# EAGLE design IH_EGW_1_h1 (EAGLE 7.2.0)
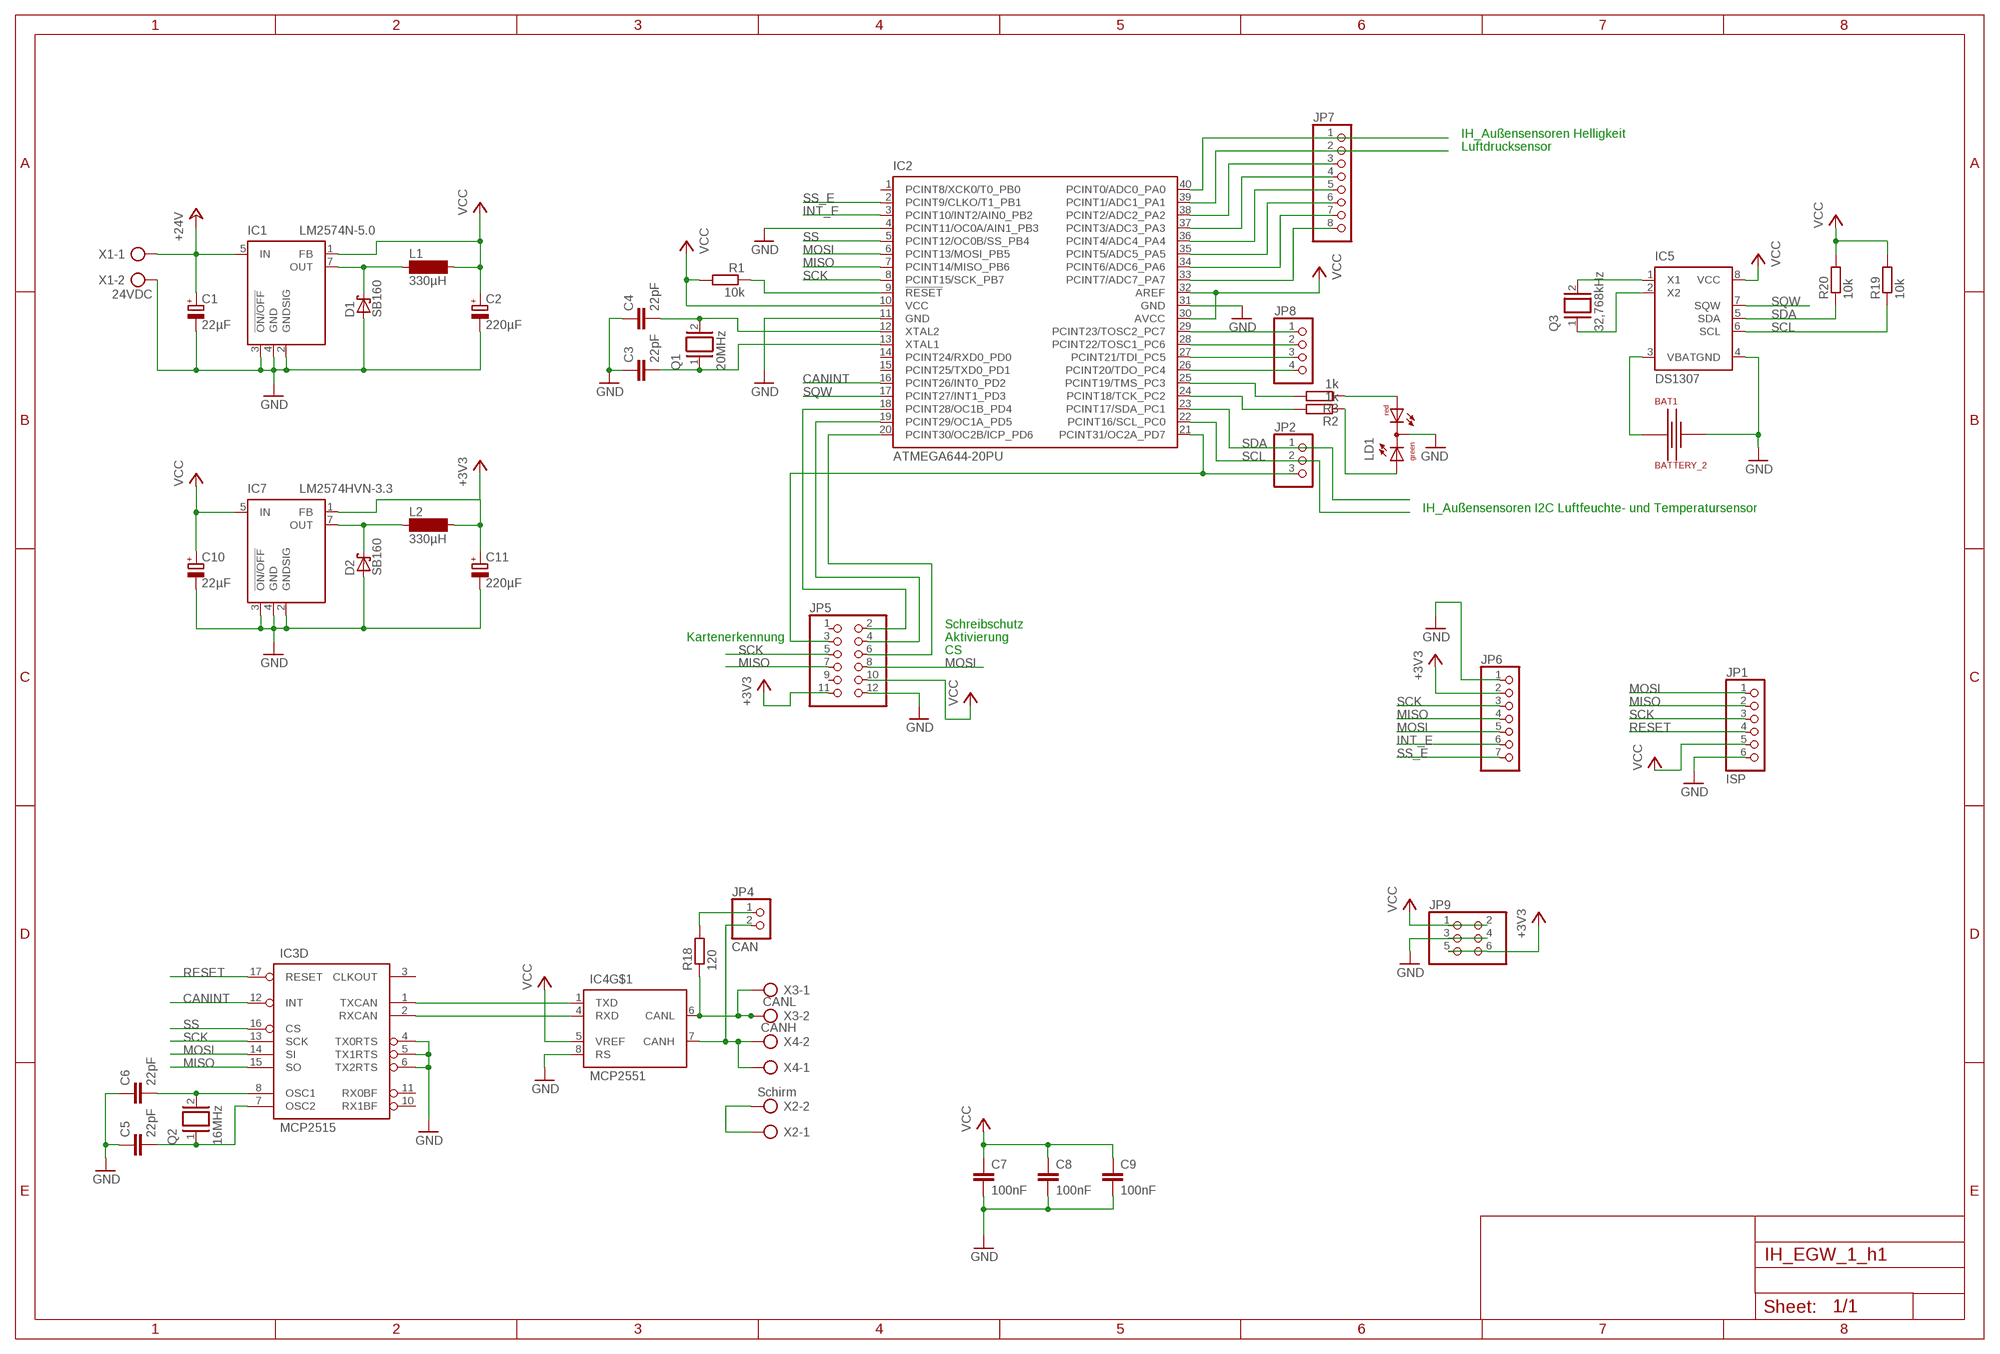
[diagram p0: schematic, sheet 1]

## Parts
BAT1  BATTERY_2  [BATTERY_2]
C1  22µF  CPOL-EUE2-5  [E2-5]
C2  220µF  CPOL-EUE3.5-8  [E3,5-8]
C3  22pF  C-EUC0805  [C0805]
C4  22pF  C-EUC0805  [C0805]
C5  22pF  C-EUC0805  [C0805]
C6  22pF  C-EUC0805  [C0805]
C7  100nF  C-EUC0805  [C0805]
C8  100nF  C-EUC0805  [C0805]
C9  100nF  C-EUC0805  [C0805]
C10  22µF  CPOL-EUE2-5  [E2-5]
C11  220µF  CPOL-EUE3.5-8  [E3,5-8]
D1  SB160  SCHOTTKY-DIODEDO35-7  [DO35-7]
D2  SB160  SCHOTTKY-DIODEDO35-7  [DO35-7]
IC1  LM2574N-5.0  [DIL08]
IC2  ATMEGA644-20PU  [DIL40]
IC3  MCP2515  MCP2515P  [DIL18]
IC4  MCP2551  MCP2551DIL8  [DIL08]
IC5  DS1307  [DIP-8]
IC7  LM2574HVN-3.3  [DIL08]
JP1  ISP  PINHD-1X6  [1X06]
JP2  PINHD-1X3  [1X03]
JP4  CAN  PINHD-1X2  [1X02]
JP5  PINHD-2X6  [2X06]
JP6  PINHD-1X7  [1X07]
JP7  PINHD-1X8  [1X08]
JP8  PINHD-1X4  [1X04]
JP9  PINHD-2X3  [2X03]
L1  330µH  SD12-1000  [SD12_1000]
L2  330µH  SD12-1000  [SD12_1000]
LD1  DUOLED-RG-C  [DUOLED-C-5MM]
Q1  20MHz  XTAL/S  [QS]
Q2  16MHz  XTAL/S  [QS]
Q3  32,768kHz  XTAL/S  [QS]
R1  10k  R-EU_R0805  [R0805]
R2  1k  R-EU_M0805  [M0805]
R3  1k  R-EU_M0805  [M0805]
R18  120  R-EU_M0805  [M0805]
R19  10k  R-EU_M0805  [M0805]
R20  10k  R-EU_M0805  [M0805]
X1  24VDC  AK300/2  [AK300/2]
X2  Schirm  AK300/2  [AK300/2]
X3  CANL  AK300/2  [AK300/2]
X4  CANH  AK300/2  [AK300/2]

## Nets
+3V3: C11.+ IC7.1(FB) JP5.11 JP6.2 JP9.5 JP9.6 L2.2
+24V: C1.+ IC1.5(IN) X1.1
CANINT: IC2.16(PCINT26/INT0_PD2) IC3.12(D:INT)
GND: BAT1.P$2(-) C1.- C2.- C3.1 C4.1 C5.1 C6.1 C7.2 C8.2 C9.2 C10.- C11.- D1.A D2.A IC1.2(GNDSIG) IC1.3(!ON/OFF) IC1.4(GND) IC2.4(PCINT11/OC0A/AIN1_PB3) IC2.11(GND) IC2.31(GND) IC3.4(D:TX0RTS) IC3.5(D:TX1RTS) IC3.6(D:TX2RTS) IC4.8(RS) IC5.4(GND) IC7.2(GNDSIG) IC7.3(!ON/OFF) IC7.4(GND) JP1.6 JP5.12 JP6.1 JP9.3 JP9.4 LD1.C X1.2
INT_E: IC2.3(PCINT10/INT2/AIN0_PB2) JP6.6
MISO: IC2.7(PCINT14/MISO_PB6) IC3.15(D:SO) JP1.2 JP5.7 JP6.4
MOSI: IC2.6(PCINT13/MOSI_PB5) IC3.14(D:SI) JP1.1 JP5.8 JP6.5
N$1: IC3.1(D:TXCAN) IC4.1(TXD)
N$2: IC3.2(D:RXCAN) IC4.4(RXD)
N$3: C6.2 IC3.8(D:OSC1) Q2.2
N$4: C5.2 IC3.7(D:OSC2) Q2.1
N$7: C4.2 IC2.12(XTAL2) Q1.2
N$8: C3.2 IC2.13(XTAL1) Q1.1
N$9: IC2.33(PCINT7/ADC7_PA7) JP7.8
N$10: IC2.34(PCINT6/ADC6_PA6) JP7.7
N$11: IC2.35(PCINT5/ADC5_PA5) JP7.6
N$12: IC2.36(PCINT4/ADC4_PA4) JP7.5
N$13: IC2.37(PCINT3/ADC3_PA3) JP7.4
N$14: IC2.38(PCINT2/ADC2_PA2) JP7.3
N$15: IC2.39(PCINT1/ADC1_PA1) JP7.2
N$16: IC4.6(CANL) R18.1 X3.1 X3.2
N$17: IC4.7(CANH) JP4.2 X4.1 X4.2
N$18: IC2.40(PCINT0/ADC0_PA0) JP7.1
N$19: IC2.29(PCINT23/TOSC2_PC7) JP8.1
N$20: IC2.20(PCINT30/OC2B/ICP_PD6) JP5.6
N$22: IC2.19(PCINT29/OC1A_PD5) JP5.4
N$23: IC2.18(PCINT28/OC1B_PD4) JP5.2
N$24: IC2.28(PCINT22/TOSC1_PC6) JP8.2
N$25: IC2.27(PCINT21/TDI_PC5) JP8.3
N$26: IC2.25(PCINT19/TMS_PC3) R3.2
N$27: D2.C IC7.7(OUT) L2.1
N$28: IC2.26(PCINT20/TDO_PC4) JP8.4
N$29: BAT1.P$1(+) IC5.3(VBAT)
N$30: IC2.21(PCINT31/OC2A_PD7) JP2.3 JP5.3
N$31: IC5.1(X1) Q3.2
N$32: IC5.2(X2) Q3.1
N$33: IC2.24(PCINT18/TCK_PC2) R2.2
N$42: LD1.AX(AG) R2.1
N$43: LD1.AR R3.1
N$44: JP4.1 R18.2
N$54: X2.1 X2.2
N$76: D1.C IC1.7(OUT) L1.1
RESET: IC2.9(!RESET) IC3.17(D:RESET) JP1.4 R1.1
SCK: IC2.8(PCINT15/SCK_PB7) IC3.13(D:SCK) JP1.3 JP5.5 JP6.3
SCL: IC2.22(PCINT16/SCL_PC0) IC5.6(SCL) JP2.2 R19.1
SDA: IC2.23(PCINT17/SDA_PC1) IC5.5(SDA) JP2.1 R20.1
SQW: IC2.17(PCINT27/INT1_PD3) IC5.7(SQW)
SS: IC2.5(PCINT12/OC0B/SS_PB4) IC3.16(D:CS)
SS_E: IC2.2(PCINT9/CLKO/T1_PB1) JP6.7
VCC: C2.+ C7.1 C8.1 C9.1 C10.+ IC1.1(FB) IC2.10(VCC) IC2.30(AVCC) IC2.32(AREF) IC4.5(VREF) IC5.8(VCC) IC7.5(IN) JP1.5 JP5.10 JP9.1 JP9.2 L1.2 R1.2 R19.2 R20.2
Unconnected: IC2.1(PCINT8/XCK0/T0_PB0) IC2.14(PCINT24/RXD0_PD0) IC2.15(PCINT25/TXD0_PD1) IC3.3(D:CLKOUT) IC3.10(D:RX1BF) IC3.11(D:RX0BF) JP5.1 JP5.9

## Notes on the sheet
- IH_Außensensoren Helligkeit
- Luftdrucksensor
- IH_Außensensoren I2C Luftfeuchte- und Temperatursensor
- Schreibschutz
- Kartenerkennung | Aktivierung
- CS

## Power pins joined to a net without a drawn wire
GND: IC3.9(P:GND) IC4.2(GND)
VCC: IC3.18(P:VCC) IC4.3(VCC)

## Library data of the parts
BAT1 = special:BATTERY_2
C1 C2 C10 C11 = rcl:CPOL-EU: POLARIZED CAPACITOR, European symbol
C3-C9 = rcl:C-EU: CAPACITOR, European symbol
D1 D2 = diode:SCHOTTKY-DIODE: Schottky Diode
IC1 IC7 = linear:LM2574?-*: SIMPLE SWITCHER 0.5A Step-Down Voltage Regulator Source: http://cache.national.com/ds/LM/LM2574.pdf
IC2 = atmel:ATMEGA644-*PU: 8-bit Microcontroller with 64K Bytes In-System Programmable Flash Auto generated by make-symbol-device-package-bsdl.ulp Rev. 34 Source: http://www.atmel.com/dyn/resources/prod_documents/doc2593.pdf; MPN: ATMEGA644-20PU; OC_FARNELL: 1288340; OC_NEWARK: 23M5060
IC3 = can:MCP2515: MC2515 Stand-Alone CAN Controller With SPI Interface, Microchip
IC4 = can:MCP2551: CAN Tranceiver Microchip
IC5 = DS1307:DS1307: DS1307 - 64×8, Serial, I2C Real Time Clock
JP1 = pinhead:PINHD-1X6: PIN HEADER
JP2 = pinhead:PINHD-1X3: PIN HEADER
JP4 = pinhead:PINHD-1X2: PIN HEADER
JP5 = pinhead:PINHD-2X6: PIN HEADER
JP6 = pinhead:PINHD-1X7: PIN HEADER
JP7 = pinhead:PINHD-1X8: PIN HEADER
JP8 = pinhead:PINHD-1X4: PIN HEADER
JP9 = pinhead:PINHD-2X3: PIN HEADER
L1 L2 = inductor-neosid:SD12: INDUCTOR; OC_FARNELL: unknown; OC_NEWARK: unknown
LD1 = led:DUOLED-RG-C: DUO LED 2 colors (red/green), 5 mm, round, common Cathode www.ligitek.com or other producers.
Q1-Q3 = special:XTAL/S: CRYSTAL
R1 R18 = rcl:R-EU_: RESISTOR, European symbol
R2 R3 R19 R20 = resistor:R-EU_: RESISTOR, European symbol
X1-X4 = con-ptr500:AK300/2: CONNECTOR; OC_FARNELL: unknown; OC_NEWARK: unknown

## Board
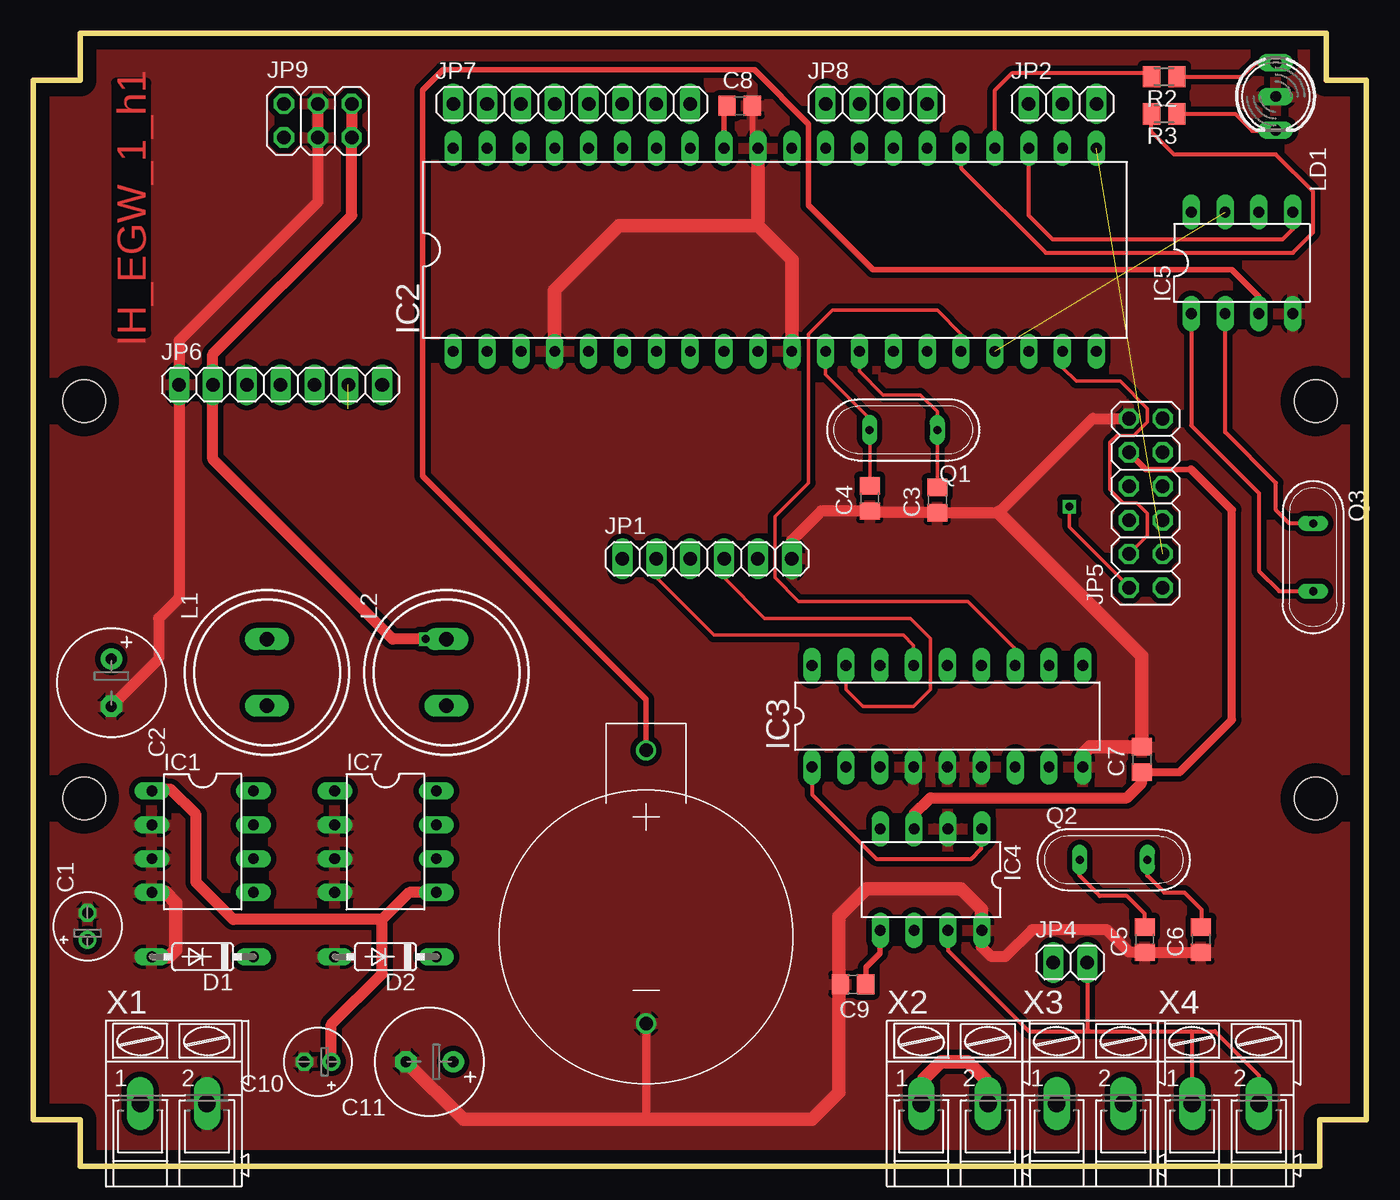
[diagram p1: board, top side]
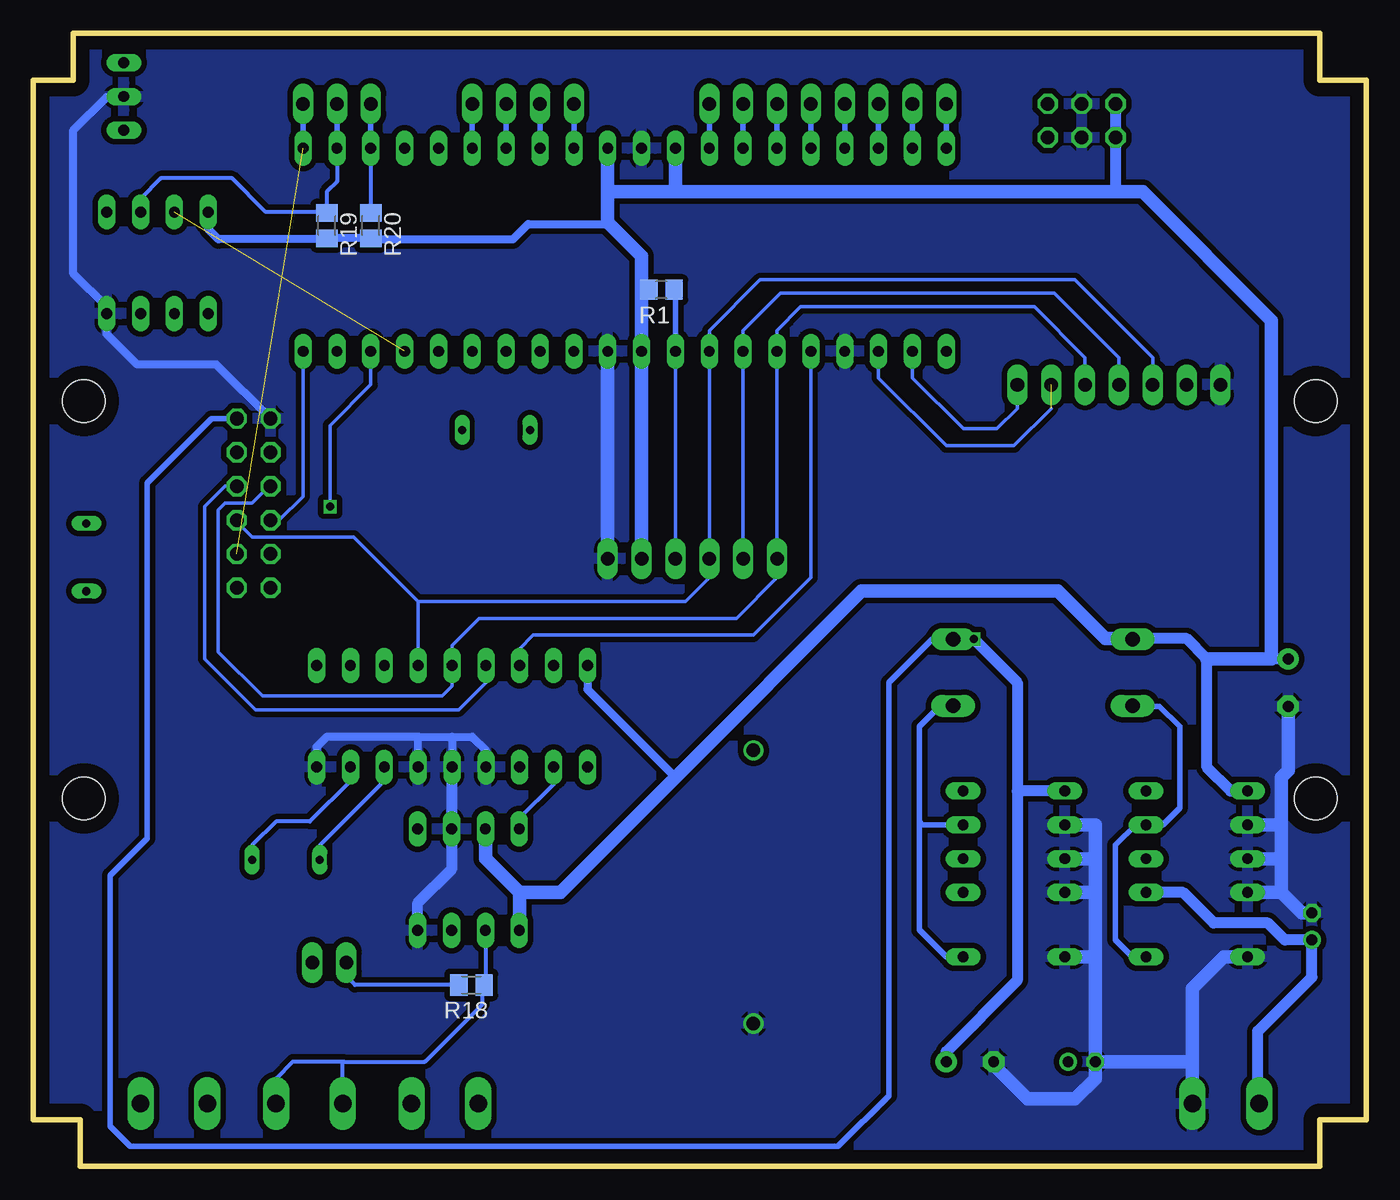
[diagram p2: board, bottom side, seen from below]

Size 100 x 85 mm. Coordinates in mm from the lower left corner, seen from the top.
Outline: 100,3.5 100,80
Outline: 0,80 0,3.5
Outline: 0,3.5 3.5,3.5 3.5,0 96.5,0 96.5,3.5 100,3.5
Outline: 0,3.5 0,81.5 3.5,81.5 3.5,85 97,85 97,81.5 100,81.5 100,3.5
Copper layers (1*16): Top 0.035mm / dielectric 1.5mm / Bottom 0.035mm
Design rules "default *": minimum track width 10mil, minimum drill 36mil, track to track 15mil, track to pad 15mil, pad to pad 10mil, via to via 10mil, smd to smd 10mil, copper to edge 40mil, drill to drill 8mil, minimum pad ring 10mil, minimum via ring 8mil, stop-mask expansion 4mil, vias tented up to drill 0mil, thermal gap 10mil
Holes 3.2 mm at 3.8,27.6 3.8,57.4 96.2,27.6 96.2,57.4

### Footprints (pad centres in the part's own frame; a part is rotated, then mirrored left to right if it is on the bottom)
BATTERY_2 = drill 1: P$1 0,0; P$2 0,20.5
E2-5 = drill 0.813 pad 1.27: + -1.016,0 | drill 0.813 pad 1.27 octagon: - 1.016,0
E3,5-8 = drill 0.813 pad 1.6: + -1.778,0 | drill 0.813 pad 1.6 octagon: - 1.778,0
C0805 = smd 1.3 x 1.5: 1 -0.95,0; 2 0.95,0
DO35-7 = drill 0.813 long: A 3.81,0; C -3.81,0
DIL08 = drill 0.813 pad 1.27 long: 1 -3.81,-3.81; 2 -1.27,-3.81; 3 1.27,-3.81; 4 3.81,-3.81; 5 3.81,3.81; 6 1.27,3.81; 7 -1.27,3.81; 8 -3.81,3.81
DIL40 = drill 0.813 long: 1 -24.13,-7.62; 2 -21.59,-7.62; 3 -19.05,-7.62; 4 -16.51,-7.62; 5 -13.97,-7.62; 6 -11.43,-7.62; 7 -8.89,-7.62; 8 -6.35,-7.62; 9 -3.81,-7.62; 10 -1.27,-7.62; 11 1.27,-7.62; 12 3.81,-7.62; 13 6.35,-7.62; 14 8.89,-7.62; 15 11.43,-7.62; 16 13.97,-7.62; 17 16.51,-7.62; 18 19.05,-7.62; 19 21.59,-7.62; 20 24.13,-7.62; 21 24.13,7.62; 22 21.59,7.62; 23 19.05,7.62; 24 16.51,7.62; 25 13.97,7.62; 26 11.43,7.62; 27 8.89,7.62; 28 6.35,7.62; 29 3.81,7.62; 30 1.27,7.62; 31 -1.27,7.62; 32 -3.81,7.62; 33 -6.35,7.62; 34 -8.89,7.62; 35 -11.43,7.62; 36 -13.97,7.62; 37 -16.51,7.62; 38 -19.05,7.62; 39 -21.59,7.62; 40 -24.13,7.62
DIL18 = drill 0.813 long: 1 -10.16,-3.81; 2 -7.62,-3.81; 3 -5.08,-3.81; 4 -2.54,-3.81; 5 0,-3.81; 6 2.54,-3.81; 7 5.08,-3.81; 8 7.62,-3.81; 9 10.16,-3.81; 10 10.16,3.81; 11 7.62,3.81; 12 5.08,3.81; 13 2.54,3.81; 14 0,3.81; 15 -2.54,3.81; 16 -5.08,3.81; 17 -7.62,3.81; 18 -10.16,3.81
DIL08' = drill 0.813 long: 1 -3.81,-3.81; 2 -1.27,-3.81; 3 1.27,-3.81; 4 3.81,-3.81; 5 3.81,3.81; 6 1.27,3.81; 7 -1.27,3.81; 8 -3.81,3.81
DIP-8 = drill 0.813 long: 1 -3.81,-3.81; 2 -1.27,-3.81; 3 1.27,-3.81; 4 3.81,-3.81; 5 3.81,3.81; 6 1.27,3.81; 7 -1.27,3.81; 8 -3.81,3.81
1X06 = drill 1.016 long: 1 -6.35,0; 2 -3.81,0; 3 -1.27,0; 4 1.27,0; 5 3.81,0; 6 6.35,0
1X03 = drill 1.016 long: 1 -2.54,0; 2 0,0; 3 2.54,0
1X02 = drill 1.016 long: 1 -1.27,0; 2 1.27,0
2X06 = drill 1.016 octagon: 1 -6.35,-1.27; 2 -6.35,1.27; 3 -3.81,-1.27; 4 -3.81,1.27; 5 -1.27,-1.27; 6 -1.27,1.27; 7 1.27,-1.27; 8 1.27,1.27; 9 3.81,-1.27; 10 3.81,1.27; 11 6.35,-1.27; 12 6.35,1.27
1X07 = drill 1.016 long: 1 -7.62,0; 2 -5.08,0; 3 -2.54,0; 4 0,0; 5 2.54,0; 6 5.08,0; 7 7.62,0
1X08 = drill 1.016 long: 1 -8.89,0; 2 -6.35,0; 3 -3.81,0; 4 -1.27,0; 5 1.27,0; 6 3.81,0; 7 6.35,0; 8 8.89,0
1X04 = drill 1.016 long: 1 -3.81,0; 2 -1.27,0; 3 1.27,0; 4 3.81,0
2X03 = drill 1.016 octagon: 1 -2.54,-1.27; 2 -2.54,1.27; 3 0,-1.27; 4 0,1.27; 5 2.54,-1.27; 6 2.54,1.27
SD12_1000 = drill 1.1 long: 1 -2.5,0; 2 2.5,0
DUOLED-C-5MM = drill 0.813 long: AR 2.54,0; AX -2.54,0; C 0,0
QS = drill 0.61 long: 1 -2.54,0; 2 2.54,0
R0805 = smd 1.3 x 1.5: 1 -0.95,0; 2 0.95,0
M0805 = smd 1.3 x 1.6: 1 -0.95,0; 2 0.95,0
AK300/2 = drill 1.321 long: 1 -2.515,0; 2 2.489,0

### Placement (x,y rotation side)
BAT1  45.98,31.2 180 top
C1  4.07,17.99 90 top
C2  5.85,36.28 270 top
C3  67.83,49.99 90 top
C4  62.75,50.11 90 top
C5  83.38,17 90 top
C6  87.61,17 90 top
C7  83.17,30.51 90 top
C8  53,79.56 0 top
C9  61.5,13.65 180 top
C10  21.34,7.83 180 top
C11  29.73,7.83 180 top
D1  12.71,15.71 180 top
D2  26.42,15.71 180 top
IC1  12.71,24.34 270 top
IC2  55.63,68.76 0 top
IC3  68.59,33.76 0 top
IC4  MCP2551  [DIL08']  67.35,21.5 180 top
IC5  90.69,67.78 0 top
IC7  26.42,24.34 270 top
JP1  50.55,45.58 0 top
JP2  77.22,79.72 0 top
JP4  77.79,15.28 0 top
JP5  83.47,49.74 90 top
JP6  18.55,58.63 0 top
JP7  40.39,79.72 0 top
JP8  63.25,79.72 0 top
JP9  21.34,78.45 0 top
L1  17.53,37.04 90 top
L2  31,37.04 90 top
LD1  93.21,80.26 270 top
Q1  65.28,55.24 180 top
Q2  81.05,22.99 0 top
Q3  96.02,45.68 270 top
R1  52.88,65.76 180 bottom
R2  84.84,81.75 180 top
R3  84.84,78.95 180 top
R18  67.13,13.59 180 bottom
R19  77.99,70.57 270 bottom
R20  74.68,70.57 270 bottom
X1  10.54,4.7 0 top
X2  69.14,4.7 0 top
X3  79.3,4.7 0 top
X4  89.46,4.7 0 top

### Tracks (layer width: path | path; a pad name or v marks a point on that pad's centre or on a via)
+3V3  (via drill 0.6)
  Top 0.813: v29.43,39.54 26.97,39.54 13.47,53.05 JP6.2 13.47,60.92 23.88,71.33 JP9.5 JP9.6
  Bottom 0.406: L2.2 32.56,39.54 35.82,36.28 35.82,5.29 39.63,1.48 92.72,1.48 94.24,3.01 94.24,21.8 91.45,24.6 91.45,51.27 86.62,56.09 JP5.11
  Bottom 0.813: C11.+ 31.5,8.6 26.17,13.93 26.17,28.15 | IC7.1 26.17,28.15 | L2.2 v29.43,39.54 26.17,36.28 26.17,28.15
+24V
  Bottom 0.813: X1.1 8.14,4.7 8.14,10.12 4.07,14.18 C1.+ 6.1,16.98 7.37,18.25 11.44,18.25 13.72,20.53 IC1.5
CANINT
  Top 0.254: IC3.12 73.67,38.82 70.11,42.38 57.41,42.38 55.63,44.16 55.63,48.73 58.17,51.27 58.17,62.44 59.95,64.22 67.83,64.22 69.6,62.44 IC2.16
GND
  Top 0.406: C9.2 60.55,15.36 60.46,15.45 | IC2.31 53.95,76.8 C8.2
  Top 0.61: BAT1.P$2 45.98,3.52
  Top 0.813: JP5.12 79.51,56.09 72.45,49.04 72.4,49.04 C3.1 62.87,49.04 C4.1 59.11,49.16 56.9,46.95 JP1.6 | C6.1 C5.1 82.22,16.05 80.53,17.74 74.94,17.74 72.91,15.71 71.89,15.71 71.13,16.47 71.13,17.66 IC4.8 | C2.- 9.41,38.06 9.41,41.11 10.93,42.63 JP6.1 10.93,61.94 21.34,72.35 JP9.3 JP9.4
  Top 1.016: IC2.31 54.36,70.57 | 54.36,70.57 56.9,68.03 IC2.11 | IC2.4 39.12,65.75 43.95,70.57 54.36,70.57 | 72.4,49.04 83.17,38.27 C7.2 79.26,31.46 78.75,30.95 IC3.9 | C11.- 32.27,3.52 45.98,3.52 58.43,3.52 60.46,5.55 60.46,15.45 60.46,18.76 62.49,20.79 69.6,20.79 71.13,19.26 71.13,17.99 | IC1.4 9.91,20.53 10.68,19.77 10.68,16.22 10.17,15.71 D1.A
  Bottom 0.406: 68.62,29.95 IC3.5
  Bottom 0.61: IC3.6 71.13,32.22 | 71.13,32.22 68.59,32.22 | 71.13,32.22 77.99,32.22 78.75,31.46 IC3.9 | 68.59,32.22 IC3.5 | 68.59,32.22 67.06,32.22 66.05,31.2 IC3.4 | LD1.C 93.25,80.22 94.5,80.22 97.04,77.68 97.04,67.02 94.5,64.48 IC5.4 94.5,62.44 92.21,60.16 86.26,60.16 JP5.12
  Bottom 0.813: 68.62,29.95 IC4.2 68.59,25.28 68.59,22.31 71.16,19.74 IC4.8
  Bottom 1.016: X1.2 13.03,7.83 | 13.03,7.83 13.03,13.36 10.68,15.71 D1.A | C10.- 13.03,7.83 | C10.- 20.33,15.96 | 20.33,15.96 20.33,20.53 | 20.33,20.53 20.33,23.07 | 20.33,23.07 20.33,25.61 IC7.2 | IC7.3 20.33,23.07 | IC7.4 20.33,20.53 | D2.A 20.58,15.71 20.33,15.96 | C2.- 5.85,29.68 6.36,29.17 6.36,25.61 | 6.36,25.61 6.36,23.07 | 6.36,23.07 6.36,20.79 | 6.36,20.79 6.36,20.53 4.83,19.01 C1.- | IC1.4 6.61,20.53 6.36,20.79 | IC1.3 6.36,23.07 | IC1.2 6.36,25.61 | C11.- 27.95,7.58 25.41,5.04 21.85,5.04 20.33,6.56 C10.- | IC2.11 JP1.6
  pour Bottom (isolate 0.406): -2.79,87.59 101.86,87.59 101.86,-2.83 -3.29,-2.83 -3.29,87.59
  pour Top (isolate 0.406): -2.28,86.83 102.37,86.83 102.37,-2.07 -1.77,-2.07 -1.77,86.57
INT_E  (1 unrouted)
  Bottom 0.254: IC2.3 36.58,59.14 31.5,54.06 26.42,54.06 23.63,56.86
MISO
  Top 0.254: JP1.2 46.74,44.16 51.06,39.84 65.29,39.84 66.05,39.08 IC3.15
  Bottom 0.254: JP1.2 IC2.7 46.74,62.7 43.95,65.49 23.38,65.49 18.55,60.67 JP6.4 | JP5.7 85.61,51.01 87.13,49.49 87.13,38.06 83.32,34.25 68.08,34.25 66.05,36.28 IC3.15
MOSI
  Bottom 0.254: JP5.8 82.3,51.01 83.57,49.74 85.61,49.74 86.11,49.24 86.11,38.57 82.81,35.27 69.35,35.27 68.59,36.03 IC3.14 68.59,39.08 66.56,41.11 47.25,41.11 44.2,44.16 JP1.1 IC2.6 44.2,62.7 42.43,64.48 24.9,64.48 21.09,60.67 JP6.5
N$1
  Top 0.305: IC3.1 58.43,27.9 63.25,23.07 70.37,23.07 71.13,23.84 71.13,25.28 IC4.1
N$2
  Bottom 0.305: IC3.2 60.97,28.66 63.51,26.12 63.51,25.34 IC4.4
N$3
  Top 0.305: Q2.2 83.59,21.82 83.57,21.8 84.84,20.53 86.37,20.53 87.64,19.26 87.64,17.98 C6.2
  Bottom 0.305: IC3.8 76.21,28.92 79.26,25.87 81.8,25.87 83.57,24.09 83.57,23 Q2.2
N$4
  Top 0.305: C5.2 83.38,18.95 82.05,20.28 80.02,20.28 78.49,21.8 78.49,22.98 Q2.1
  Bottom 0.305: IC3.7 73.67,28.92 78.49,24.09 78.49,22.98 | 78.49,22.57 78.49,22.98 | 78.49,22.98 Q2.1
N$6  (via drill 0.6)
  other vias: 77.73,49.49
N$7
  Top 0.254: C4.2 Q1.2 62.75,55.25 62.75,56.09 59.44,59.4 IC2.12
N$8
  Top 0.254: IC2.13 61.98,59.65 63.76,57.87 66.56,57.87 67.83,56.6 67.83,55.25 Q1.1 67.82,50.95 C3.2
N$9
  Bottom 0.406: JP7.8 IC2.33
N$10
  Bottom 0.406: JP7.7 IC2.34
N$11
  Bottom 0.406: JP7.6 IC2.35
N$12
  Bottom 0.406: JP7.5 IC2.36
N$13
  Bottom 0.406: JP7.4 IC2.37
N$14
  Bottom 0.406: JP7.3 IC2.38
N$15
  Bottom 0.406: JP7.2 IC2.39
N$16
  Bottom 0.305: IC4.6 66.08,13.7 R18.1 66.3,13.48 66.3,12.15 70.62,7.83 76.72,7.83 | X3.1 76.78,7.76 76.72,7.83 | 76.72,7.83 80.53,7.83 81.8,6.56 X3.2
N$17
  Top 0.305: IC4.7 68.62,16.18 74.68,10.12 79.26,10.12 | 79.26,10.12 86.88,10.12 | 86.88,10.12 88.65,10.12 91.96,6.82 X4.2 | X4.1 86.94,10.05 86.88,10.12 | JP4.2 79.06,10.31 79.26,10.12
N$18
  Bottom 0.406: JP7.1 IC2.40
N$19
  Bottom 0.406: JP8.1 IC2.29
N$20
  Bottom 0.254: JP5.6 81.54,48.47 79.76,50.25 IC2.20
N$22
  Top 0.254: IC2.19 77.22,59.9 78.24,58.89 81.54,58.89 83.57,56.86 83.57,55.84 82.56,54.82 81.29,54.82 80.78,54.32 80.78,50.76 81.8,49.74 82.81,49.74 83.57,48.98 83.57,47.31 JP5.4
N$23  (via drill 0.6)
  Top 0.254: JP5.2 82.2,43.5 77.73,47.97 v77.73,49.49
  Bottom 0.254: v77.73,49.49 77.73,55.59 74.68,58.63 IC2.18
N$24
  Bottom 0.406: JP8.2 IC2.28
N$25
  Bottom 0.406: JP8.3 IC2.27
N$26
  Top 0.305: IC2.25 69.6,74.89 75.95,68.54 94.5,68.54 96.02,70.06 96.02,73.11 93.23,75.91 85.61,75.91 83.89,77.62 R3.2
N$27
  Bottom 0.406: D2.C 31.5,15.71 33.54,17.74 33.54,25.87 | 33.54,25.87 33.54,32.98 32.01,34.5 31.04,34.5 L2.1 | IC7.7 33.28,25.61 33.54,25.87
N$28
  Bottom 0.406: JP8.4 IC2.26
N$29
  Top 0.406: IC5.3 91.96,65.24 89.92,67.27 63,67.27 58.17,72.1 58.17,78.19 54.11,82.26 30.74,82.26 29.22,80.73 29.22,51.78 45.98,35.01 BAT1.P$1
N$30  (1 unrouted)
  Bottom 0.406: IC2.21 JP2.3
N$31
  Top 0.305: IC5.1 86.88,55.59 91.96,50.51 91.96,44.66 93.48,43.14 Q3.2
N$32
  Top 0.305: Q3.1 94.24,48.22 93.23,49.24 93.23,51.27 89.42,55.08 IC5.2
N$33
  Top 0.305: IC2.24 72.14,80.73 73.41,82 83.64,82 R2.2
N$42
  Top 0.305: R2.1 90.69,81.75 91.7,82.76 93.17,82.76 LD1.AX
N$43
  Top 0.305: R3.1 90.18,78.95 91.45,77.68 93.17,77.68 LD1.AR
N$44
  Bottom 0.305: R18.2 75.87,13.59 76.46,14.18 76.46,15.22 JP4.1
N$54
  Top 1.016: X2.1 66.81,4.7 66.81,6.56 68.08,7.83 70.11,7.83 71.38,6.56 71.38,4.95 X2.2
N$76
  Bottom 0.406: L1.1 17.49,34.5 15.5,34.5 13.98,32.98 13.98,26.88 15.25,25.61 IC1.7 17.28,25.61 18.8,24.09 18.8,16.98 17.53,15.71 D1.C
RESET
  Top 0.254: IC3.17 60.97,35.77 62.24,34.5 66.05,34.5 67.32,35.77 67.32,39.58 65.79,41.11 54.87,41.11 51.82,44.16 JP1.4
  Bottom 0.254: IC2.9 JP1.4
  Bottom 0.406: 51.93,61.24 IC2.9 51.82,65.65 R1.1
SCK
  Bottom 0.254: 71.13,42.38 51.06,42.38 49.28,44.16 JP1.3 IC2.8 49.28,62.7 45.47,66.51 21.85,66.51 16.01,60.67 JP6.3 | JP5.5 84.74,48.37 83.57,47.2 75.95,47.2 71.13,42.38 | IC3.13 71.13,42.38
SCL
  Bottom 0.305: IC2.22 77.22,73.87 77.99,73.11 R19.1 78.05,71.59 82.56,71.59 85.1,74.13 90.43,74.13 91.96,72.6 IC5.6
  Bottom 0.406: JP2.2 IC2.22
SDA
  Top 0.305: IC5.5 94.5,70.32 93.73,69.56 76.46,69.56 74.68,71.33 IC2.23
  Bottom 0.305: IC2.23 R20.1
  Bottom 0.406: JP2.1 IC2.23
SQW  (1 unrouted)
SS
  Bottom 0.254: IC3.16 63.51,38.82 62.49,39.84 45.98,39.84 41.66,44.16 IC2.5
SS_E
  Bottom 0.254: JP6.7 26.17,56.86 27.69,55.33 30.23,55.33 34.04,59.14 IC2.2
VCC
  Top 0.406: 86.88,52.28 83.47,52.28 JP5.10 | C9.1 62.45,14.9 63.51,15.96 63.51,17.66 IC4.5 | C8.1 51.82,79.34 IC2.32
  Top 0.61: C7.1 86,29.56 89.92,33.49 89.92,49.24 86.88,52.28
  Top 0.813: C10.+ 22.36,10.63 26.17,14.44 26.17,18.5 | 30.74,20.53 IC7.5 28.2,20.53 26.17,18.5 | 26.17,18.5 14.99,18.5 12.2,21.3 12.2,26.38 10.29,28.28 9.53,28.28 9.41,28.15 IC1.1 | 66.05,25.34 66.05,26.38 67.32,27.65 82.05,27.65 83.17,28.76 C7.1
  Top 1.016: IC4.3 66.05,25.34
  Bottom 0.406: 54.1,66.01 54.36,65.75 | R1.2 54.09,65.49 54.36,65.49
  Bottom 0.61: 56.78,70.7 62.87,70.7 64.02,69.56 74.62,69.56 R20.2 R19.2 78.05,69.56 86.11,69.56 86.88,70.32 IC5.8 | IC3.18 58.43,35.77 51.82,29.17
  Bottom 0.813: C2.+ 7.12,38.06 | L1.2 17.49,39.58 17.03,39.58 13.47,39.58 11.95,38.06 11.95,29.93 10.17,28.15 IC1.1 | JP9.2 JP9.1 18.8,73.11
  Bottom 1.016: 11.95,38.06 7.12,38.06 7.12,63.46 16.77,73.11 18.8,73.11 51.82,73.11 | JP1.5 IC2.10 54.36,65.49 54.36,65.75 54.36,68.29 56.78,70.7 56.9,70.83 56.9,72.86 | 56.9,72.86 IC2.30 | IC2.32 51.82,73.11 | 56.9,72.86 56.65,73.11 51.82,73.11 | 63.51,20.53 66.08,23.11 IC4.3 | 63.51,20.53 63.51,17.72 IC4.5 | 17.03,39.58 19.57,39.58 23.12,43.14 37.85,43.14 51.82,29.17 60.46,20.53 63.51,20.53

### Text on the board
Top: IH_EGW_1_h1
